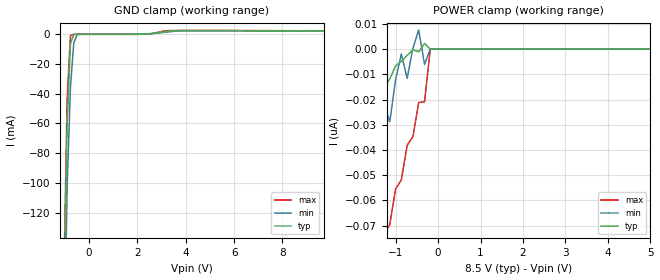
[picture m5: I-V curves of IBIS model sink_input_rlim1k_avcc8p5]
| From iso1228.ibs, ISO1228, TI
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|   Model sink_input_rlim1k_avcc8p5
[Model] sink_input_rlim1k_avcc8p5
Model_type Input
Vinl =  5.100V
Vinh =  6.000V
C_comp   0.859pF   0.874pF   1.06pF
[Model Spec]
Vinh   6.000V   5.700V   6.400V
Vinl   5.100V   4.700V   5.300V
[Temperature Range]   27.000   150   -40
[Voltage Range]   8.500V   8.500V   8.500V
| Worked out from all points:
|   GND clamp passes 1 mA (typ) near -0.66 V on its own axis
[GND_clamp]
|Voltage   I(typ)   I(min)   I(max)
-8.5V     -12.68A    -12.59A    -12.74A
-1.045V   -181mA     -225.2mA   -164.1mA
-909mV    -60.35mA   -101.6mA   -42.73mA
-773mV    -6.234mA   -35.31mA   -784.6uA
-636mV    -85.21uA   -5.931mA   -2.405uA
-500mV    -1.063uA   -254.8uA   -728.8nA
2.364V    132.2uA    294.9uA    113.4uA
3.182V    1.768mA    1.469mA    2.328mA
3.864V    2.473mA    2.348mA    2.584mA
17V       1.944mA    1.851mA    2.039mA
[POWER_clamp]
|Voltage   I(typ)   I(min)   I(max)
-8.5V     -1.169uA   -1.993uA   -1.035uA
-2.364V   -77.9nA    -144.2nA   -156.8nA
-1.818V   -40.6nA    -71.17nA   -112.5nA
-1.545V   -26.52nA   -56.19nA   -92.51nA
-1.273V   -15.24nA   -21.99nA   -73.59nA
-1.136V   -11.82nA   -28.82nA   -69.52nA
-864mV    -4.865nA   -1.972nA   -51.86nA
-727mV    -2.501nA   -11.6nA    -38.16nA
-455mV    -1.058nA   7.604nA    -21.19nA
-318mV    2.191nA    -6.124nA   -20.89nA
-182mV    0A         0A         0A
5V        0A         0A         0A
